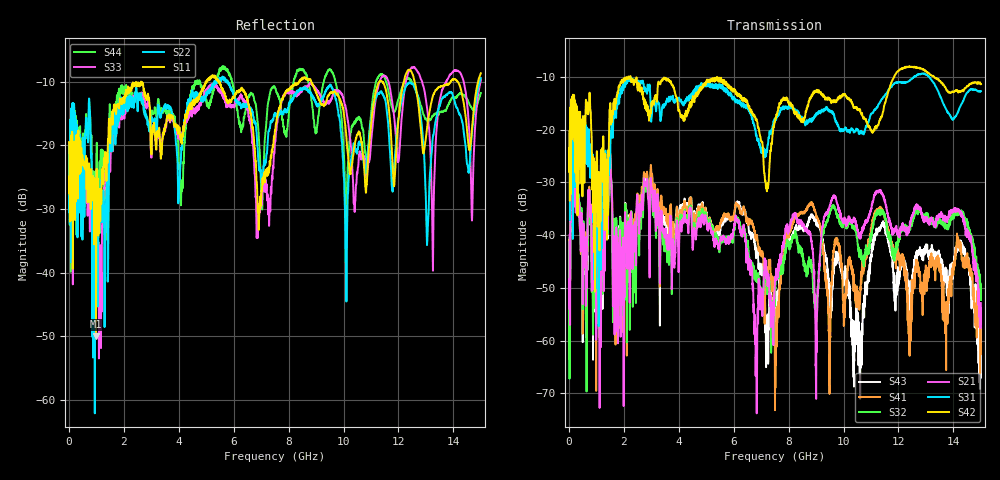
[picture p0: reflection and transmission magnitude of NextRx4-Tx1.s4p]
! FILE: N:\QM 2007\Prüfprotokolle\Highspeed\Konfektionierte Ltg\L45593-D106\D30\8216\0002\Next  Platine 2\NextRx4-Tx1.s4p
# MHz S DB R 50.00
! FREQ  S11  S12  S13  S14
!  S21  S22  S23  S24
!  S31  S32  S33  S34
!  S41  S42  S43  S44
!  DB  ANG  DB  ANG  DB  ANG  DB  ANG
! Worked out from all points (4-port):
!   2999 points, 10 MHz to 15 GHz, reference 50 ohm
!   strongest paths, dB at 10 MHz, 3.755 GHz, 7.505 GHz, 11.26 GHz, 15 GHz:
!     S42: -23.6, -11.5, -18.4, -19.2, -11.4
!     S31: -24.8, -13.8, -18.4, -15.5, -12.7
!     S21: -48.4, -47.1, -48.8, -31.6, -52.9
!     S32: -43.1, -48.1, -51.0, -35.8, -52.3
!     S41: -41.0, -40.9, -73.2, -35.2, -60.7
!     S43: -43.8, -42.2, -54.8, -39.0, -58.3
!   lowest |S11| = -49.9 dB at 990 MHz (marker M1), VSWR 1.01, Z = 50 - j0.318 ohm
!   |S11| at or under -10 dB: start of sweep to 5.008 GHz; 5.49 GHz to 8.378 GHz (2.888 GHz wide, 41.6 % of centre); 8.826 GHz to 11.3 GHz (2.476 GHz wide, 24.6 % of centre)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
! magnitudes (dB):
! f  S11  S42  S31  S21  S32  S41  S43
! 10 MHz  -19.5  -23.6  -24.8  -48.4  -43.1  -41.0  -43.8
! 990 MHz  -49.9  -31.2  -37.3  -47.0  -44.2  -44.8  -43.9
! 2.19 GHz  -10.9  -10.3  -10.8  -39.2  -42.9  -38.7  -39.6
! 6.82 GHz  -24.1  -18.1  -21.1  -59.8  -47.5  -40.9  -44.4
! 9.53 GHz  -11.7  -14.5  -16.7  -33.9  -35.4  -53.5  -52.2
! 10.1 GHz  -18.4  -13.8  -19.8  -38.3  -38.8  -49.5  -46.8
! 15 GHz  -8.7  -11.4  -12.7  -52.9  -52.3  -60.7  -58.3
